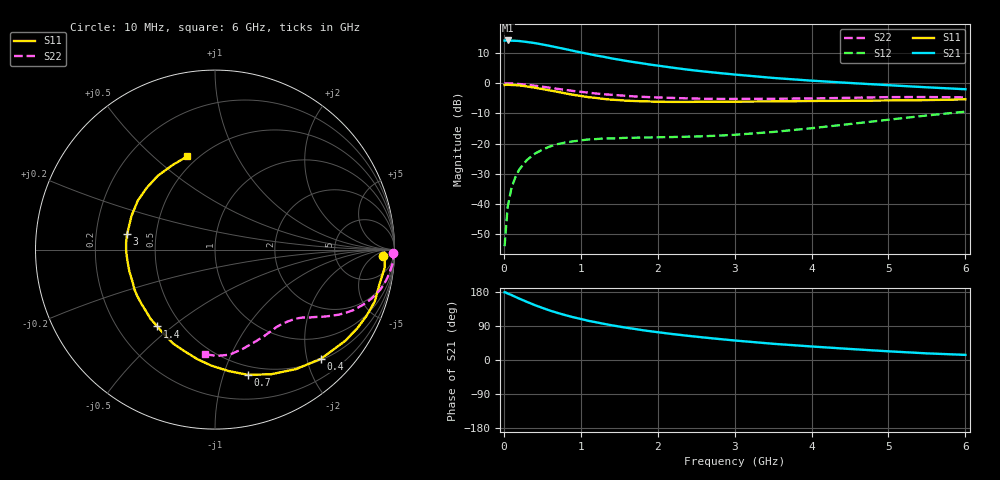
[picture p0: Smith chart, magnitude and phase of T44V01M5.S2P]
! Infineon Technologies  Discrete & RF Semiconductors
! BFR182T
! Si NPN RF Bipolar Junction Transistor in SC75
! VCE = 4 V  IC = 1.5 mA
! Common Emitter S-Parameters:  October  1999
# GHz  S  MA  R  50
!  f  S11  S21  S12  S22
! GHz  MAG  ANG  MAG  ANG  MAG  ANG  MAG  ANG
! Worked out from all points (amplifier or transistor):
!   36 points, 10 MHz to 6 GHz, reference 50 ohm
!   highest |S21| = 14.2 dB at 50 MHz (marker M1)
!   |S21| within 3 dB of that: start of sweep to 824.9 MHz
!   unconditionally stable (mu >= 1): 2.193 GHz to 4.449 GHz
!   at 250 MHz: K = 0.12, MSG = 20.4 dB, |S12| = -27.0 dB
!   at 1.4 GHz: K = 0.69, MSG = 13.3 dB, |S12| = -18.3 dB
!   at 6 GHz: K = 0.82, MSG = 3.7 dB, |S12| = -9.4 dB
!   S11 on the Smith chart (normalised r, x): 10 MHz: 23, -14; 400 MHz: 0.52, -2.27; 700 MHz: 0.42, -1.21; 1.4 GHz: 0.37, -0.44; 3 GHz: 0.34, +0.08; 6 GHz: 0.44, +0.65
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0.01  0.9378 -2.2  5.106 178.6  0.002 83.6  0.9902 -1.2
0.02  0.9451 -1.0  5.109 178.6  0.003 99.9  0.9999 -1.0
0.05  0.9508 -6.1  5.134 175.5  0.009 90.2  0.9952 -2.4
0.1  0.937 -11.5  5.091 171.4  0.0186 85.8  0.9912 -4.8
0.2  0.9216 -23.6  5.024 162.1  0.0372 77.2  0.9736 -9.3
0.3  0.8865 -34.9  4.843 153.4  0.0535 70.6  0.9477 -13.6
0.4  0.848 -45.8  4.651 145.0  0.0678 64.5  0.9141 -17.4
0.5  0.8043 -55.9  4.406 137.6  0.0794 59.5  0.8796 -20.5
0.6  0.7614 -65.8  4.164 130.4  0.09 55.5  0.8445 -23.4
0.7  0.7218 -75.2  3.919 124.2  0.0983 51.7  0.8094 -25.8
0.9  0.6457 -92.1  3.461 113.0  0.1093 45.3  0.7477 -29.5
1.1  0.5897 -107.2  3.073 103.4  0.1174 41.4  0.6997 -32.4
1.4  0.5353 -126.9  2.589 91.7  0.1222 37.4  0.646 -35.9
1.6  0.5139 -139.2  2.341 84.9  0.1253 36.4  0.6185 -37.7
1.8  0.5044 -149.5  2.144 78.8  0.1264 36.5  0.5967 -40.0
2.2  0.4923 -165.7  1.813 68.3  0.1289 38.3  0.5724 -44.1
2.6  0.4952 -179.1  1.572 59.4  0.1328 41.8  0.5554 -49.0
3  0.4972 170.0  1.399 51.5  0.1403 46.3  0.5509 -53.6
3.5  0.5017 158.0  1.229 42.8  0.1563 52.0  0.5545 -60.5
4.5  0.513 137.9  1.013 29.1  0.2114 58.8  0.5753 -74.8
5.5  0.5269 116.9  0.859 17.5  0.2932 58.4  0.5926 -88.9
6  0.542 106.6  0.798 13.5  0.3394 55.6  0.5854 -95.3
